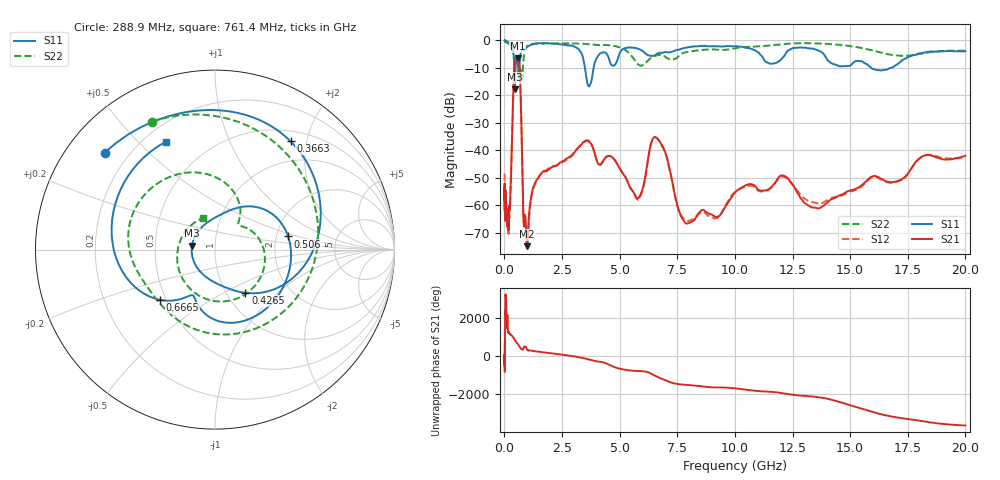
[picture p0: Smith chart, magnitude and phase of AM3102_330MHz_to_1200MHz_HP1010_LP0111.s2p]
! Date/Time: Tue, Sep 11, 2018 5:19 PM
! Network Analyzer: Agilent Technologies E8362B Rev: A.07.50.63
! Sweep from 0.010 to 20.000 GHz, 1601 Points, Sweep Type: LOG
! Power Supply: 4.949 V, 0.001 A
# Hz S DB R 50
!freq MagS11 AngS11 MagS21 AngS21 MagS12 AngS12 MagS22 AngS22
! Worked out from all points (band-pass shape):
!   1601 points, 10 MHz to 20 GHz, reference 50 ohm
!   highest |S21| = -6.42 dB at 586.3 MHz (marker M1); lowest = -74.8 dB at 993.4 MHz (marker M2)
!   |S21| within 3 dB of the highest: 428.5 MHz to 651.5 MHz (223 MHz wide, 41.3 % of centre)
!   lowest |S11| = -17.7 dB at 451.5 MHz (marker M3), VSWR 1.30, Z = 38.6 + j1.77 ohm
!   |S11| at or under -10 dB: 424.9 MHz to 481 MHz (56.08 MHz wide, 12.4 % of centre); 3.497 GHz to 3.871 GHz (373.7 MHz wide, 10.1 % of centre); 15.91 GHz to 16.76 GHz (840.7 MHz wide, 5.15 % of centre)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
!   |S22| runs from -14.5 to -0.2 dB; largest |S21 - S12| = 0.0088
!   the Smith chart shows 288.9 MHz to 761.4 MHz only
!   S11 on the Smith chart (normalised r, x): 288.9 MHz: 0.11, +0.37; 366.3 MHz: 0.66, +1.73; 426.5 MHz: 1.22, -0.65; 506 MHz: 2.33, +0.41; 666.5 MHz: 0.46, -0.31; 761.4 MHz: 0.28, +0.61
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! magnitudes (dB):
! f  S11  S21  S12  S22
! 10 MHz  0.0  -55.6  -48.8  -0.2
! 35.55 MHz  0.0  -63.9  -62.9  -0.4
! 126.4 MHz  -0.4  -65.7  -63.0  -0.9
! 187.5 MHz  -0.8  -66.8  -69.2  -1.1
! 288.9 MHz  -1.7  -49.4  -49.4  -2.0
! 366.3 MHz  -2.7  -24.8  -24.8  -4.6
! 426.5 MHz  -10.6  -9.7  -9.8  -7.0
! 447.2 MHz  -17.6  -7.6  -7.6  -7.4
! 451.5 MHz  -17.7  -7.3  -7.4  -7.4
! 506 MHz  -7.7  -6.8  -6.8  -6.0
! 586.3 MHz  -8.6  -6.4  -6.6  -9.7
! 666.5 MHz  -7.6  -11.5  -11.5  -11.9
! 761.4 MHz  -3.6  -39.0  -39.1  -14.5
! 833.3 MHz  -3.3  -66.0  -65.1  -6.6
! 993.4 MHz  -2.3  -74.8  -73.4  -1.9
! 1.59 GHz  -1.1  -48.5  -48.4  -1.0
! 3.107 GHz  -2.6  -39.8  -40.0  -1.1
! 3.599 GHz  -15.4  -36.5  -36.3  -1.3
! 5.652 GHz  -2.7  -56.0  -56.1  -7.1
! 6.58 GHz  -5.1  -35.2  -35.4  -5.5
! 7.995 GHz  -2.4  -66.4  -65.5  -4.1
! 20 GHz  -3.9  -41.9  -42.5  -3.7
